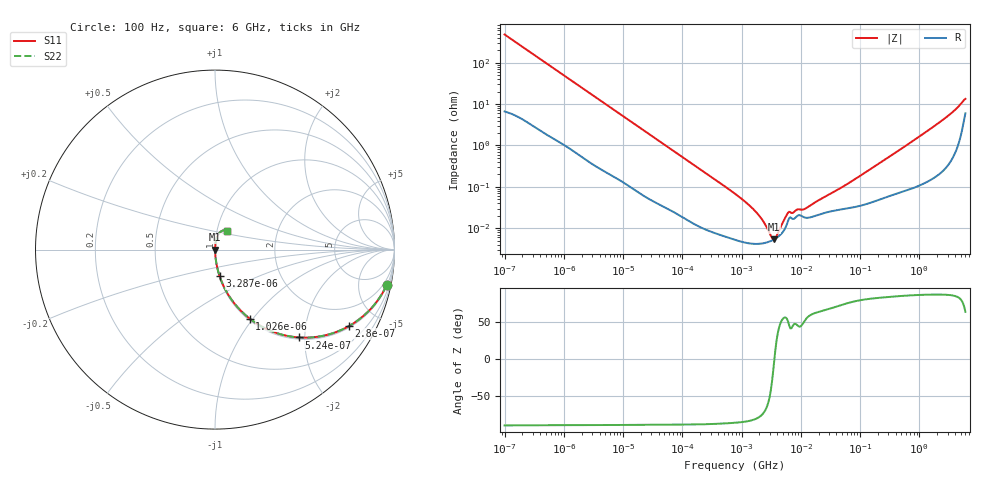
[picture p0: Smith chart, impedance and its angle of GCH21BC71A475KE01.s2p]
!Murata Part Number: GCH21BC71A475KE01
!These Parameters are Measured in Series Mode Connection
!Data Generated on Jun 19, 2026
!  o--ll--o
!Port1  Port2
!  o------o
!Operation Temp=25[degC], DC Bias Voltage=0[V]
!Freq. Start=100[Hz] Stop=6[GHz] 401[Steps]
# Hz S RI R 50
!Freq.(Hz) S11(Real) S11(Imag) S21(Real) S21(Imag) S12(Real) S12(Imag) S22(Real) S22(Imag)
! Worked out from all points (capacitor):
!   401 points, 100 Hz to 6 GHz, reference 50 ohm
!   read as one part in series: C = 3.31 uF near 109 Hz
!   lowest |Z| = 5.41 mohm at 3.55 MHz (marker M1)
!   series resonance near 3.582 MHz, so ESL is about 600 pH
!   S11 on the Smith chart (normalised r, x): 100 Hz: 1.13, -9.58; 280 Hz: 1.06, -3.47; 524 Hz: 1.04, -1.87; 1.026 kHz: 1.02, -0.96; 3.287 kHz: 1.01, -0.30; 6 GHz: 1.12, +0.24
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100  0.9557 -0.1989  0.0443 0.1989  0.0443 0.1989  0.9557 -0.1989
164  0.8926 -0.3012  0.1074 0.3012  0.1074 0.3012  0.8926 -0.3012
280  0.7465 -0.426  0.2535 0.426  0.2535 0.426  0.7465 -0.426
524  0.4662 -0.4894  0.5338 0.4894  0.5338 0.4894  0.4662 -0.4894
1026  0.1929 -0.3843  0.8071 0.3843  0.8071 0.3843  0.1929 -0.3843
2008  0.0623 -0.2314  0.9377 0.2314  0.9377 0.2314  0.0623 -0.2314
3287  0.0258 -0.1481  0.9742 0.1481  0.9742 0.1481  0.0258 -0.1481
9204  0.00442 -0.055  0.9956 0.055  0.9956 0.055  0.00442 -0.055
40335  0.000545 -0.0129  0.9995 0.0129  0.9995 0.0129  0.000545 -0.0129
774597  5.29e-05 -0.000679  0.9999 0.000679  0.9999 0.000679  5.29e-05 -0.000679
1658239  4.2e-05 -0.000266  1 0.000266  1 0.000266  4.2e-05 -0.000266
2713602  4.58e-05 -8.9e-05  1 8.9e-05  1 8.9e-05  4.58e-05 -8.9e-05
3549919  5.4e-05 -2.8e-06  0.9999 2.8e-06  0.9999 2.8e-06  5.4e-05 -2.8e-06
4440638  6.8e-05 7.13e-05  0.9999 -7.13e-05  0.9999 -7.13e-05  6.8e-05 7.13e-05
5809218  0.000124 0.000173  0.9999 -0.000173  0.9999 -0.000173  0.000124 0.000173
6353432  0.000175 0.000179  0.9998 -0.000179  0.9998 -0.000179  0.000175 0.000179
1.137099e7  0.000184 0.000222  0.9998 -0.000222  0.9998 -0.000222  0.000184 0.000222
1.555665e7  0.000189 0.000332  0.9998 -0.000332  0.9998 -0.000332  0.000189 0.000332
5.960426e7  0.000301 0.00111  0.9997 -0.00111  0.9997 -0.00111  0.000301 0.00111
3.124326e8  0.000625 0.00531  0.9994 -0.00531  0.9994 -0.00531  0.000625 0.00531
2.34314e9  0.0037 0.0385  0.9963 -0.0385  0.9963 -0.0385  0.0037 0.0385
6e9  0.0681 0.1053  0.9319 -0.1053  0.9319 -0.1053  0.0681 0.1053
